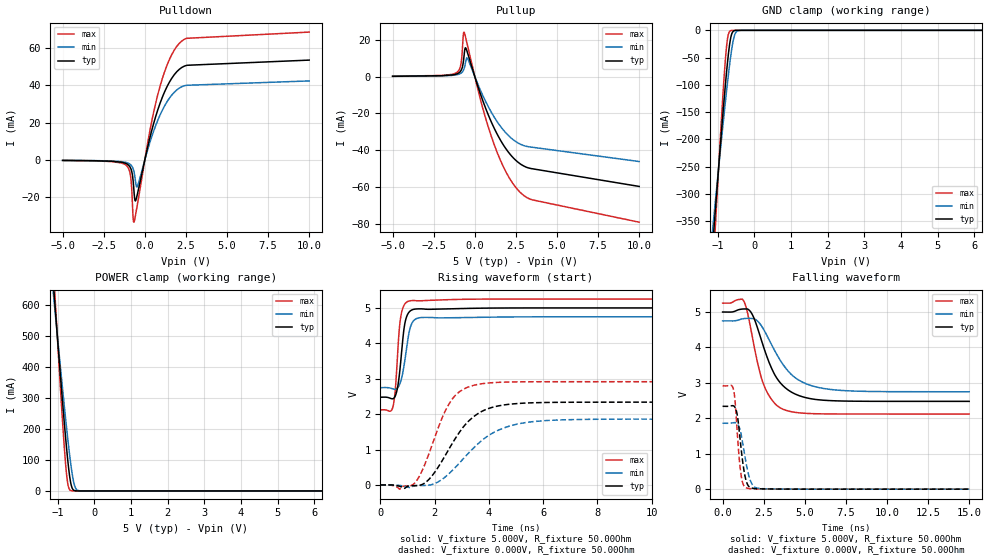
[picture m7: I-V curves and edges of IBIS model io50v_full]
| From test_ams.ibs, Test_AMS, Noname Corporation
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[Model]   io50v_full
Model_type   I/O
Vinl = 800.000mV
Vinh = 2.000V
Vmeas = 1.400V
Vref = 1.400V
Cref = 0.000F
Rref = 50.000Ohm
|   typ   min   max
C_comp   3.000pF   2.000pF   4.000pF
[Voltage Range]   5.000V   4.750V   5.250V
[Temperature Range]   50.0   100.0   0.0
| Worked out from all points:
|   slope of the pulldown table from 0 to 0.75 V, typ, clamps not added: 29.2 ohm
|   slope of the pullup table from 0 to 0.75 V, typ, clamps not added: 39 ohm
|   GND clamp passes 1 mA (typ) near -0.56 V on its own axis
|   POWER clamp passes 1 mA (typ) near -0.54 V on its own axis
|   falling waveform, V_fixture 5.000V, R_fixture 50.00Ohm: 20-80 % time 1.39ns typ, 1.73ns min, 1.02ns max; typ from 5 V to 2.48 V
|   rising waveform, V_fixture 5.000V, R_fixture 50.00Ohm: 20-80 % time 208ps typ, 249ps min, 173ps max; typ from 2.48 V to 5 V
|   rising waveform, V_fixture 0.000V, R_fixture 50.00Ohm: 20-80 % time 1.25ns typ, 1.59ns min, 928ps max; typ from 0 V to 2.34 V
|   falling waveform, V_fixture 0.000V, R_fixture 50.00Ohm: 20-80 % time 365ps typ, 451ps min, 288ps max; typ from 2.34 V to 0 V
[Pulldown]
|   Voltage   I(typ)   I(min)   I(max)
-5V       -207.1uA   -171.2uA   -248.8uA
-1.13V    -1.927mA   -1.335mA   -2.852mA
-860mV    -4.389mA   -2.516mA   -9.027mA
-710mV    -11.07mA   -4.645mA   -31mA
-670mV    -15.23mA   -5.818mA   -33.25mA
-575mV    -21.91mA   -10.83mA   -29.94mA
-445mV    -18.01mA   -13.98mA   -23.51mA
265mV     10.33mA    8.149mA    13.57mA
790mV     26.82mA    21.25mA    34.93mA
1.37V     39.56mA    31.41mA    51.13mA
2.085V    48.39mA    38.37mA    62.25mA
10V       53.44mA    42.3mA     68.42mA
[GND Clamp]
|   Voltage   I(typ)   I(min)   I(max)
-5V       -4.027A    -3.186A    -5.543A
-1.13V    -390.7mA   -361.3mA   -444.8mA
-1.1V     -363.9mA   -340.4mA   -407.5mA
-1.06V    -328.4mA   -312.7mA   -358mA
-885mV    -177.6mA   -194mA     -151.1mA
-785mV    -97.87mA   -129.4mA   -51.4mA
-720mV    -52.41mA   -89.83mA   -11.61mA
-640mV    -13.05mA   -46.25mA   -566.3uA
-575mV    -1.921mA   -19.1mA    -34.84uA
-520mV    -281.6uA   -5.975mA   -3.374uA
-345mV    -531.1nA   -33.11uA   -5.618nA
10V       0A         0A         0A
[Pullup]
|   Voltage   I(typ)   I(min)   I(max)
-5V       149.8uA    122.3uA    183uA
-1.115V   1.394mA    953.8uA    2.1mA
-845mV    3.186mA    1.803mA    6.687mA
-660mV    10.77mA    4.082mA    24.18mA
-570mV    15.65mA    7.386mA    21.72mA
-440mV    12.84mA    9.88mA     16.84mA
340mV     -9.372mA   -7.373mA   -12.34mA
1.035V    -25.27mA   -19.83mA   -33.28mA
1.84V     -38.53mA   -30.1mA    -50.84mA
2.665V    -46.8mA    -36.26mA   -62.03mA
3.52V     -50.13mA   -38.44mA   -67.04mA
10V       -59.71mA   -46.16mA   -79.14mA
[POWER Clamp]
|   Voltage   I(typ)   I(min)   I(max)
-5V       7.053A     5.738A     9.247A
-1.11V    658.2mA    629.4mA    708.7mA
-1.08V    611.4mA    591.9mA    646.6mA
-1.055V   572.7mA    560.8mA    595.2mA
-885mV    316.1mA    353.3mA    259.7mA
-780mV    169.5mA    231.1mA    84.52mA
-715mV    90.19mA    159.9mA    18.72mA
-640mV    24.84mA    86.19mA    1.081mA
-575mV    3.782mA    36.36mA    69.66uA
-525mV    671.4uA    13.17mA    8.338uA
-340mV    886.9nA    56.68uA    6.759nA
10V       0A         0A         0A
[Ramp]
R_load = 50.00Ohm
|   typ   min   max
dV/dt_r   1.403V/1.248ns   1.116V/1.589ns   1.750V/927.496ps
dV/dt_f   1.513V/1.385ns   1.201V/1.726ns   1.878V/1.020ns
[Falling Waveform]
V_fixture = 5.000V
V_fixture_min = 4.750V
V_fixture_max = 5.250V
R_fixture = 50.00Ohm
|   Time   V(typ)   V(min)   V(max)
0s        5V         4.75V      5.25V
1.275ns   5.086V     4.812V     5.318V
1.5ns     5.086V     4.82V      5.009V
1.8ns     4.935V     4.817V     4.318V
2.45ns    4.075V     4.545V     3.013V
3.1ns     3.294V     3.97V      2.46V
3.65ns    2.931V     3.536V     2.262V
4.65ns    2.64V      3.074V     2.155V
6.25ns    2.507V     2.834V     2.124V
15ns      2.478V     2.748V     2.121V
[Rising Waveform]
V_fixture = 5.000V
V_fixture_min = 4.750V
V_fixture_max = 5.250V
R_fixture = 50.00Ohm
|   Time   V(typ)   V(min)   V(max)
0s        2.478V     2.748V     2.121V
475ps     2.438V     2.712V     2.232V
550ps     2.507V     2.704V     2.654V
625ps     2.705V     2.732V     3.504V
750ps     3.451V     2.919V     4.723V
900ps     4.536V     3.488V     5.106V
1.05ns    4.87V      4.258V     5.192V
1.225ns   4.959V     4.634V     5.209V
1.55ns    4.972V     4.73V      5.204V
15ns      5V         4.75V      5.25V
[Rising Waveform]
V_fixture = 0.000V
V_fixture_min = 0.000V
V_fixture_max = 0.000V
R_fixture = 50.00Ohm
|   Time   V(typ)   V(min)   V(max)
0s        30.4nV     275.4nV    27.1nV
725ps     -39.43mV   -14.24mV   -118.1mV
1.275ns   -18.96mV   -21.14mV   58.71mV
1.825ns   183.8mV    -1.581mV   947.9mV
2.55ns    1.038V     331.3mV    2.307V
2.925ns   1.496V     626.4mV    2.636V
3.45ns    1.933V     1.053V     2.816V
4.375ns   2.236V     1.555V     2.899V
5.7ns     2.323V     1.794V     2.915V
15ns      2.339V     1.861V     2.916V
[Falling Waveform]
V_fixture = 0.000V
V_fixture_min = 0.000V
V_fixture_max = 0.000V
R_fixture = 50.00Ohm
|   Time   V(typ)   V(min)   V(max)
0s        2.339V     1.861V     2.916V
675ps     2.348V     1.876V     2.784V
775ps     2.293V     1.876V     2.392V
875ps     2.134V     1.855V     1.715V
1.1ns     1.259V     1.605V     479.5mV
1.25ns    679.3mV    1.221V     141.7mV
1.45ns    211.2mV    684.9mV    36.33mV
1.775ns   33.16mV    154mV      12.26mV
2.25ns    10.64mV    20.44mV    6.216mV
15ns      30.4nV     275.4nV    27.1nV
